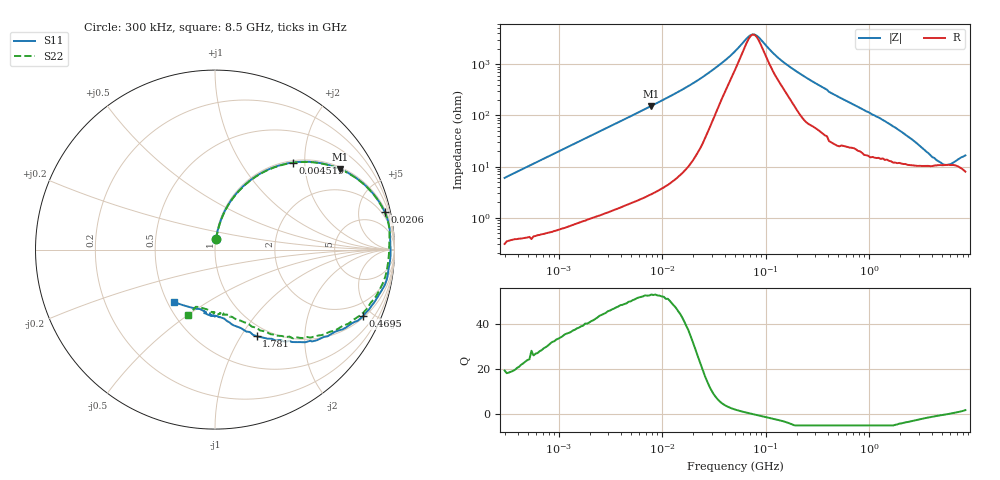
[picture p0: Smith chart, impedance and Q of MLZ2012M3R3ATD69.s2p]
! S-Parameter Data Generated by TDK Corporation
! Copyright(C) 2020 TDK Corporation.
! All Rights Reserved.
! TDK P/N: MLZ2012M3R3ATD69 (Inductor)
! Property: L=3.3uH at 2MHz
! Size(LxWxT): 2x1.25x1.25mm
! Model Type: s2p (Touchstone File Format Version 1.0)
! Frequency: DC=Yes Start=0.3MHz Stop=8500MHz 225points Log-sweep
! Model Generated on Apr. 9, 2020
! Port Assignments:
!  1 ---@@@--- 2
! Applicable Conditions:
!  Temperature = 25 degC
!  DC Bias Current = 0 A
!  Small Signal Operation
! Terms and conditions regarding TDK Simulation Models
! (1)This simulation model is being provided solely for informational purposes. Please refer to the specifications of the products in terms of detailed characteristics of such products.
! (2)In no event shall TDK Corporation of any of its subsidiaries be liable for any loss or damage arising, directly or indirectly,
!  From any information contained in this simulation model, including, but not limited to loss or damages arising from any inaccuracies, omissions or errors in connection with such information.
! (3)Any and all copyrights on this simulation model are owned by TDK Corporation.
!  Duplication or redistribution of this simulation model without prior written permission from TDK Corporation is prohibited.
! (4)This simulation model is subject to any modification or change without any prior notice.
! (5)Neither TDK Corporation nor any of its subsidiaries shall make any warranty, express or implied,
!  Including but not limited to the correctness, implied warranties of merchantability and fitness for a particular purpose with respect to this simulation models.
! (6)The use of this simulation model shall be deemed to have consented to the terms and conditions hereof.
# Hz S MA R 50
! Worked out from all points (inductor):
!   224 points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, 300 kHz to 8.5 GHz, reference 50 ohm
!   read as one part in series: L = 3.17 uH near 314.1 kHz
!   highest Q = 53.1 at 7.846 MHz (marker M1), where L = 3.1 uH
!   self-resonance near 75.94 MHz
!   S11 on the Smith chart (normalised r, x): 300 kHz: 1.01, +0.12; 4.519 MHz: 1.04, +1.75; 20.6 MHz: 1.33, +8.92; 469.5 MHz: 1.09, -4.41; 1.781 GHz: 0.87, -1.17; 8.5 GHz: 0.54, -0.37
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300000  0.06065 83.9  0.9962 -3.4  0.9937 -3.3  0.06009 83.7
752368.3  0.1462 79.8  0.984 -8.5  0.9838 -8.3  0.1461 79.7
1721110  0.3164 70.2  0.94 -18.5  0.94 -18.4  0.3162 70.0
2725608  0.4637 61.1  0.8747 -27.7  0.875 -27.5  0.4635 60.9
4519427  0.6515 48.1  0.7441 -40.8  0.7445 -40.6  0.6514 48.0
7846373  0.8285 32.9  0.5429 -56.1  0.543 -56.0  0.8284 32.7
9430415  0.8713 28.2  0.4724 -60.8  0.4726 -60.6  0.8712 28.0
2.060362e7  0.9683 12.5  0.2184 -75.6  0.2185 -75.5  0.968 12.4
5.167171e7  0.9772 2.4  0.05218 -60.4  0.05224 -60.2  0.9724 2.2
6.808408e7  0.9779 0.5  0.02841 -26.4  0.02843 -26.2  0.9706 0.2
7.815234e7  0.9784 -0.5  0.02574 7.0  0.02577 7.2  0.9699 -0.8
1.420669e8  0.974 -5.3  0.08252 65.8  0.08259 66.0  0.9662 -5.4
2.831228e8  0.9573 -13.6  0.2064 68.8  0.2065 69.0  0.9447 -13.5
4.69456e8  0.9034 -24.2  0.3565 59.9  0.3566 60.1  0.8914 -23.9
8.935346e8  0.7589 -41.8  0.5681 41.9  0.5683 42.1  0.7496 -39.7
1.551304e9  0.5765 -59.4  0.7277 23.4  0.7278 23.6  0.5789 -54.9
1.78071e9  0.5354 -64.3  0.7597 18.3  0.7601 18.6  0.5302 -59.0
2.572272e9  0.4345 -76.2  0.8188 4.7  0.8193 5.0  0.4215 -70.1
3.890506e9  0.3701 -88.4  0.8427 -10.4  0.842 -10.0  0.3663 -83.1
6.450987e9  0.3534 -98.3  0.8378 -29.4  0.8374 -29.1  0.3324 -103.7
7.404957e9  0.3447 -107.0  0.8415 -35.8  0.8418 -35.4  0.3365 -108.6
8.5e9  0.3719 -128.1  0.8312 -44.2  0.8332 -43.8  0.3954 -112.1
